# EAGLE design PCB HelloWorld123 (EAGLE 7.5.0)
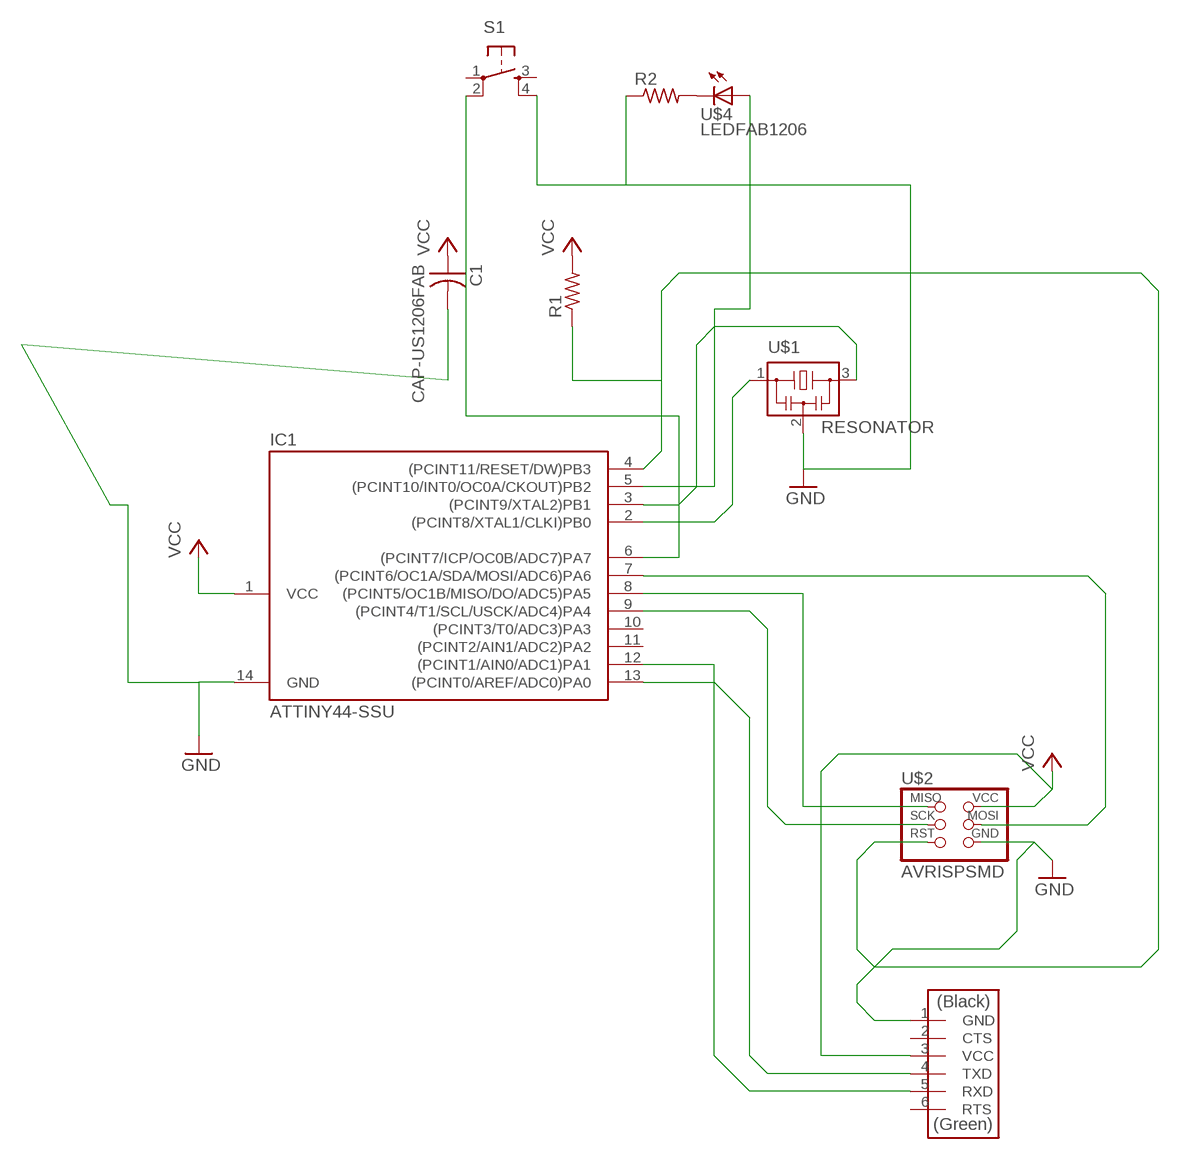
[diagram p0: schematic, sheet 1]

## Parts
C1  CAP-US1206FAB  [C1206FAB]
IC1  ATTINY44-SSU  [SOIC14]
R1  RES-US1206FAB  [R1206FAB]
R2  RES-US1206FAB  [R1206FAB]
S1  6MM_SWITCH6MM_SWITCH  [6MM_SWITCH]
U$1  RESONATOR  [EFOBM]
U$2  AVRISPSMD  [2X03SMD]
U$3  FTDI-SMD-HEADER  [1X06SMD]
U$4  LEDFAB1206  [LED1206FAB]

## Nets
GND: C1.2 IC1.14(GND) R2.1 S1.4(S1) U$1.2 U$2.6(GND) U$3.1(GND)
N$1: IC1.7((PCINT6/OC1A/SDA/MOSI/ADC6)PA6) U$2.4(MOSI)
N$2: IC1.3((PCINT9/XTAL2)PB1) U$1.3
N$3: IC1.2((PCINT8/XTAL1/CLKI)PB0) U$1.1
N$4: IC1.5((PCINT10/INT0/OC0A/CKOUT)PB2) U$4.1(A)
N$5: IC1.9((PCINT4/T1/SCL/USCK/ADC4)PA4) U$2.3(SCK)
N$6: IC1.4((PCINT11/RESET/DW)PB3) R1.1 U$2.5(RST)
N$7: IC1.8((PCINT5/OC1B/MISO/DO/ADC5)PA5) U$2.1(MISO)
N$8: IC1.13((PCINT0/AREF/ADC0)PA0) U$3.4(TXD)
N$9: IC1.12((PCINT1/AIN0/ADC1)PA1) U$3.5(RXD)
N$10: R2.2 U$4.2(C)
N$11: IC1.6((PCINT7/ICP/OC0B/ADC7)PA7) S1.2(P1)
VCC: C1.1 IC1.1(VCC) R1.2 U$2.2(VCC) U$3.3(VCC)
Unconnected: IC1.10((PCINT3/T0/ADC3)PA3) IC1.11((PCINT2/AIN1/ADC2)PA2) S1.1(P) S1.3(S) U$3.2(CTS) U$3.6(RTS)

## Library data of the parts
C1 = fab:CAP-US
IC1 = fab:ATTINY44
R1 R2 = fab:RES-US: Resistor (US Symbol)
S1 = fab:6MM_SWITCH: OMRON SWITCH
U$1 = fab:RESONATOR
U$2 = fab:AVRISP
U$3 = fab:FTDI-SMD-HEADER
U$4 = fab:LED: LED

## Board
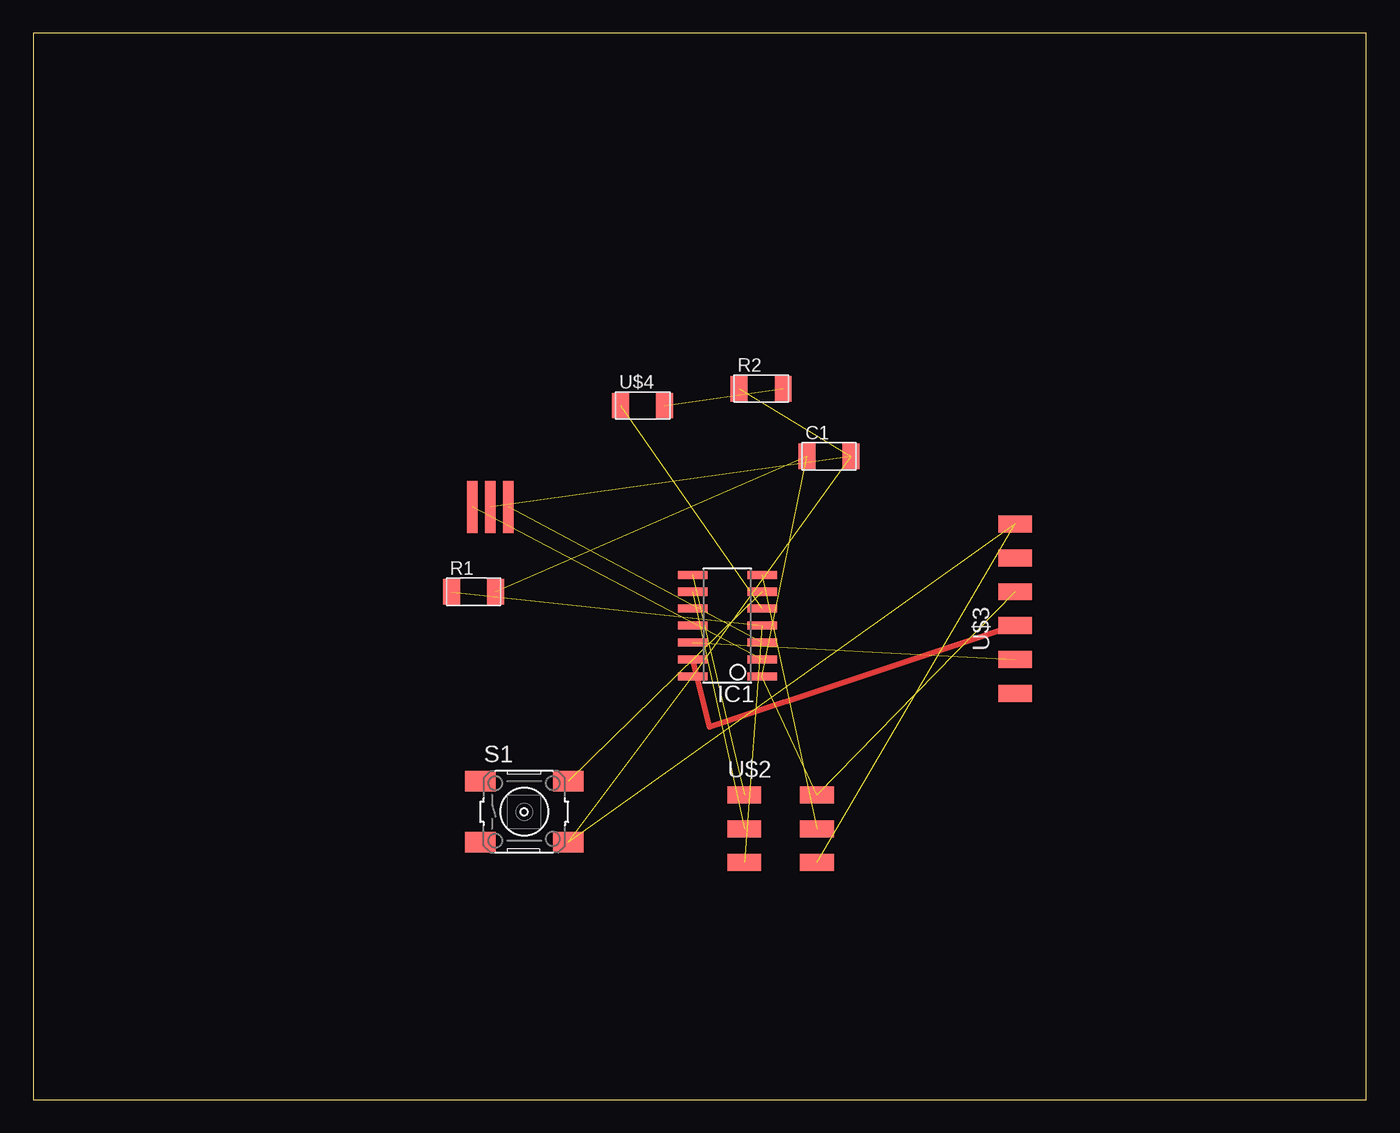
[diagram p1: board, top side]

Size 100 x 80 mm. Coordinates in mm from the lower left corner, seen from the top.
Outline: 0,0 100,0 100,80 0,80 0,0
Copper layers (1*16): Top 0.035mm / dielectric 1.5mm / Bottom 0.035mm
Design rules "default": minimum track width 10mil, minimum drill 24mil, track to track 8mil, track to pad 8mil, pad to pad 8mil, via to via 8mil, smd to smd 8mil, copper to edge 40mil, drill to drill 8mil, minimum pad ring 10mil, minimum via ring 8mil, stop-mask expansion 4mil, vias tented up to drill 0mil, thermal gap 10mil

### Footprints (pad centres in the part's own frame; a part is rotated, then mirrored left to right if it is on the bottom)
C1206FAB = smd 1.27 x 1.905: 1 -1.651,0; 2 1.651,0
SOIC14 = smd 0.61 x 2.21: 1 -3.81,-2.603; 2 -2.54,-2.603; 3 -1.27,-2.603; 4 0,-2.603; 5 1.27,-2.603; 6 2.54,-2.603; 7 3.81,-2.603; 8 3.81,2.603; 9 2.54,2.603; 10 1.27,2.603; 11 0,2.603; 12 -1.27,2.603; 13 -2.54,2.603; 14 -3.81,2.603
R1206FAB = smd 1.27 x 1.905: 1 -1.651,0; 2 1.651,0
6MM_SWITCH = smd 2.286 x 1.524: 1 -3.302,2.286; 2 3.302,2.286; 3 -3.302,-2.286; 4 3.302,-2.286
EFOBM = smd 0.8 x 3.9: 1 -1.35,0; 2 0,0; 3 1.35,0
2X03SMD = smd 2.54 x 1.27: 1 -2.54,2.54; 2 2.92,2.54; 3 -2.54,0; 4 2.92,0; 5 -2.54,-2.54; 6 2.92,-2.54
1X06SMD = smd 2.54 x 1.27: 1 0,6.35; 2 0,3.81; 3 0,1.27; 4 0,-1.27; 5 0,-3.81; 6 0,-6.35
LED1206FAB = smd 1.27 x 1.905: 1 -1.651,0; 2 1.651,0

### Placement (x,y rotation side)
C1  59.69,48.26 0 top
IC1  52.07,35.56 90 top
R1  33.02,38.1 0 top
R2  54.61,53.34 0 top
S1  36.83,21.59 0 top
U$1  34.29,44.45 0 top
U$2  55.88,20.32 0 top
U$3  73.66,36.83 0 top
U$4  45.72,52.07 0 top

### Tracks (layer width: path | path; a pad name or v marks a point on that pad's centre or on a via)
GND  (6 unrouted)
N$1  (1 unrouted)
N$2  (1 unrouted)
N$3  (1 unrouted)
N$4  (1 unrouted)
N$5  (1 unrouted)
N$6  (2 unrouted)
N$7  (1 unrouted)
N$8
  Top 0.406: U$3.4 50.74,27.94 IC1.13
N$9  (1 unrouted)
N$10  (1 unrouted)
N$11  (1 unrouted)
VCC  (4 unrouted)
